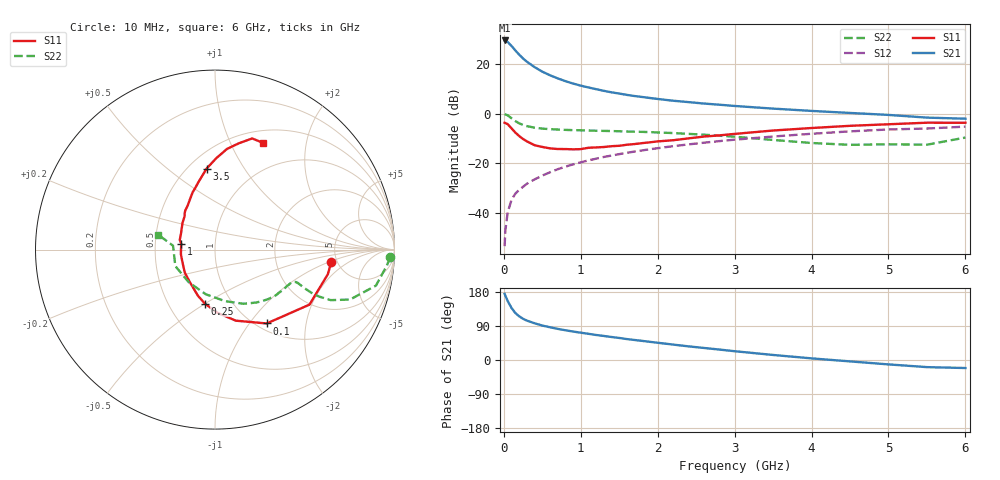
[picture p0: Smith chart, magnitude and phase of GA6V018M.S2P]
! Infineon Technologies  Discrete & RF Semiconductors
! BF775
! Si NPN RF Bipolar Junction Transistor in SOT23
! VCE = 6 V  IC = 18 mA
! Common Emitter S-Parameters:  May  1996
# GHz  S  MA  R  50
!  f  S11  S21  S12  S22
! GHz  MAG  ANG  MAG  ANG  MAG  ANG  MAG  ANG
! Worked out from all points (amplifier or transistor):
!   36 points, 10 MHz to 6 GHz, reference 50 ohm
!   highest |S21| = 29.5 dB at 10 MHz (marker M1)
!   |S21| within 3 dB of that: start of sweep to 121.1 MHz
!   unconditionally stable (mu >= 1): 446.7 MHz to 2.831 GHz
!   at 250 MHz: K = 0.82, MSG = 25.9 dB, |S12| = -29.6 dB
!   at 1.4 GHz: K = 1.10, MAG = 10.8 dB, |S12| = -17.0 dB
!   at 6 GHz: K = 0.92, MSG = 1.6 dB, |S12| = -5.3 dB
!   S11 on the Smith chart (normalised r, x): 10 MHz: 4.46, -1.09; 100 MHz: 1.11, -1.22; 250 MHz: 0.75, -0.50; 1 GHz: 0.68, +0.05; 3.5 GHz: 0.61, +0.70; 6 GHz: 0.64, +1.33
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0.01  0.6516 -6.2  29.88 174.6  0.0021 87.5  0.9768 -2.5
0.02  0.6435 -12.3  29.45 169.5  0.0044 80.8  0.9617 -5.3
0.05  0.6093 -30.2  27.88 155.7  0.0101 77.3  0.919 -12.6
0.1  0.5024 -55.0  23.12 137.3  0.0181 70.2  0.8022 -20.3
0.15  0.4125 -73.7  18.72 123.9  0.0242 65.5  0.7033 -23.6
0.2  0.351 -88.2  15.44 115.3  0.0289 66.1  0.6347 -24.3
0.25  0.3063 -100.5  12.94 108.8  0.0332 65.8  0.5876 -24.1
0.3  0.2742 -110.3  11.12 103.9  0.0383 66.9  0.5571 -23.6
0.4  0.2289 -127.8  8.642 96.9  0.0469 68.1  0.5182 -22.6
0.5  0.2116 -142.7  6.998 90.9  0.0559 69.3  0.496 -21.9
0.6  0.198 -153.7  5.921 86.4  0.0652 69.5  0.484 -21.9
0.7  0.1921 -164.7  5.128 82.2  0.075 69.6  0.4751 -22.3
0.8  0.1918 -172.3  4.506 78.5  0.0846 69.3  0.4679 -22.8
1  0.1911 170.0  3.66 72.1  0.1036 68.9  0.459 -24.5
1.1  0.2036 164.6  3.358 69.1  0.1133 68.2  0.4542 -25.7
1.3  0.2108 153.5  2.873 63.4  0.1329 66.9  0.4462 -28.2
1.6  0.2346 140.4  2.378 55.2  0.1612 64.4  0.4336 -32.7
2.2  0.2891 121.7  1.814 40.7  0.2193 58.7  0.4034 -43.4
3.5  0.454 95.9  1.257 13.3  0.3434 43.7  0.293 -78.8
4.5  0.5649 83.2  1.028 -3.7  0.4366 30.9  0.2334 -129.0
5.5  0.653 71.5  0.827 -18.8  0.498 15.7  0.2347 174.7
6  0.6519 66.0  0.787 -21.2  0.5442 11.6  0.3273 165.3
